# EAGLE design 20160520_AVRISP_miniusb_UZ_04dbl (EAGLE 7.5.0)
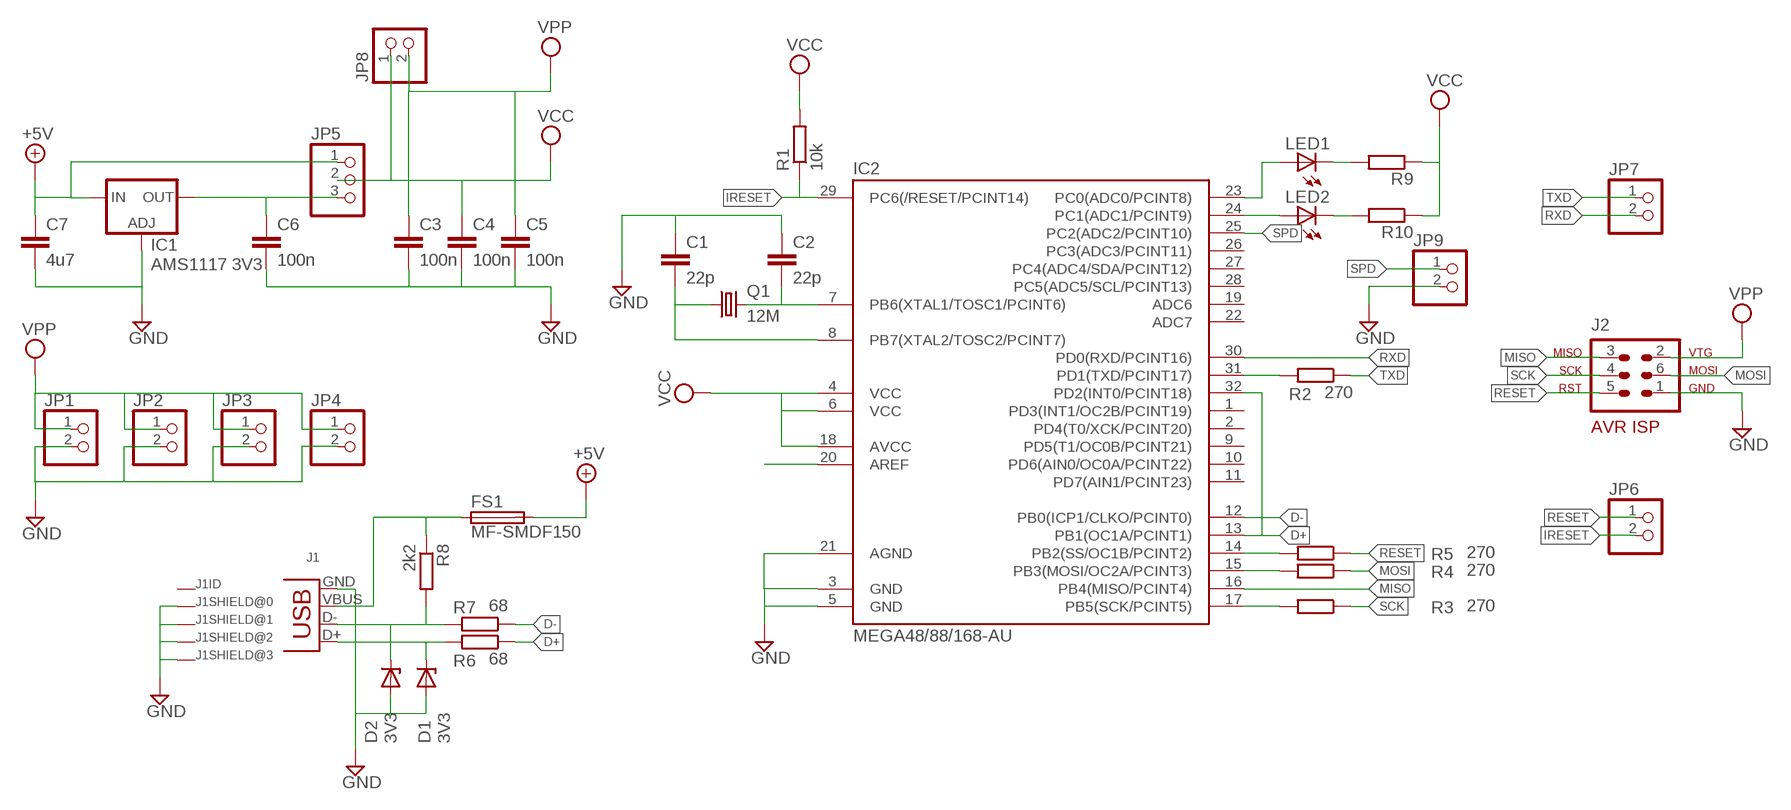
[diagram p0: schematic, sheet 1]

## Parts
C1  22p  C-EUC0805  [C0805]
C2  22p  C-EUC0805  [C0805]
C3  100n  C-EUC0805  [C0805]
C4  100n  C-EUC0805  [C0805]
C5  100n  C-EUC0805  [C0805]
C6  100n  C-EUC0805  [C0805]
C7  4u7  C-EUC1206  [C1206]
D1  3V3  ZENER-DIODESOD80C  [SOD80C]
D2  3V3  ZENER-DIODESOD80C  [SOD80C]
FS1  MF-SMDF150  [MF-SMDF050]
IC1  AMS1117 3V3  LD117AS33TR  [SOT223]
IC2  MEGA48/88/168-AU  [TQFP32-08]
J1  MINIUSB_SHIELD  [USB-MB-S2]
J2  AVR-ISP-6SPARKFUN  [SIL06]
JP1  PINHD-1X2  [1X02]
JP2  PINHD-1X2  [1X02]
JP3  PINHD-1X2  [1X02]
JP4  PINHD-1X2  [1X02]
JP5  PINHD-1X3  [1X03]
JP6  PINHD-1X2  [1X02]
JP7  PINHD-1X2  [1X02]
JP8  PINHD-1X2  [1X02]
JP9  PINHD-1X2  [1X02]
LED1  LEDCHIP-LED0805  [CHIP-LED0805]
LED2  LEDCHIP-LED0805  [CHIP-LED0805]
Q1  12M  CRYSTALHC49U-V  [HC49U-V]
R1  10k  R-EU_M0805  [M0805]
R2  270  R-EU_M0805  [M0805]
R3  270  R-EU_M0805  [M0805]
R4  270  R-EU_M0805  [M0805]
R5  270  R-EU_M0805  [M0805]
R6  68  R-EU_M0805  [M0805]
R7  68  R-EU_M0805  [M0805]
R8  2k2  R-EU_M0805  [M0805]
R9  R-EU_M0805  [M0805]
R10  R-EU_M0805  [M0805]

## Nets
+5V: C7.1 FS1.2 IC1.3(IN) JP5.1
D+: IC2.13(PB1(OC1A/PCINT1)) IC2.32(PD2(INT0/PCINT18)) R6.1
D-: IC2.12(PB0(ICP1/CLKO/PCINT0)) R7.1
GND: C1.1 C2.1 C3.2 C4.2 C5.2 C6.2 C7.2 D1.A D2.A IC1.1(ADJ) IC2.3(GND) IC2.5(GND) IC2.21(AGND) J1.GND J1.P$1(P) J1.P$2(P) J1.P$3(P) J1.P$4(P) J2.1(GND) JP1.2 JP2.2 JP3.2 JP4.2 JP9.2
IRESET: IC2.29(PC6(/RESET/PCINT14)) JP6.2 R1.1
LED1: LED1.C R9.2
MISO: IC2.16(PB4(MISO/PCINT4)) J2.3(MISO)
MOSI: J2.6(MOSI) R4.1
N$1: C2.2 IC2.7(PB6(XTAL1/TOSC1/PCINT6)) Q1.2
N$2: C1.2 IC2.8(PB7(XTAL2/TOSC2/PCINT7)) Q1.1
N$3: IC2.23(PC0(ADC0/PCINT8)) LED1.A
N$5: IC2.24(PC1(ADC1/PCINT9)) LED2.A
N$6: LED2.C R10.2
N$7: FS1.1 J1.VBUS R8.1
N$9: D2.C J1.D- R7.2 R8.2
N$10: D1.C J1.D+ R6.2
N$13: IC2.20(AREF)
N$16: IC2.31(PD1(TXD/PCINT17)) R2.2
N$17: IC2.14(PB2(SS/OC1B/PCINT2)) R5.2
N$18: IC2.15(PB3(MOSI/OC2A/PCINT3)) R4.2
N$19: IC2.17(PB5(SCK/PCINT5)) R3.2
N$22: C6.1 IC1.4(OUT) JP5.3
RESET: J2.5(RST) JP6.1 R5.1
RXD: IC2.30(PD0(RXD/PCINT16)) JP7.2
SCK: J2.4(SCK) R3.1
SPD: IC2.25(PC2(ADC2/PCINT10)) JP9.1
TXD: JP7.1 R2.1
VCC: C4.1 IC2.4(VCC) IC2.6(VCC) IC2.18(AVCC) JP5.2 JP8.1 R1.2 R9.1 R10.1
VPP: C3.1 C5.1 J2.2(VTG) JP1.1 JP2.1 JP3.1 JP4.1 JP8.2
Unconnected: IC2.1(PD3(INT1/OC2B/PCINT19)) IC2.2(PD4(T0/XCK/PCINT20)) IC2.9(PD5(T1/OC0B/PCINT21)) IC2.10(PD6(AIN0/OC0A/PCINT22)) IC2.11(PD7(AIN1/PCINT23)) IC2.19(ADC6) IC2.22(ADC7) IC2.26(PC3(ADC3/PCINT11)) IC2.27(PC4(ADC4/SDA/PCINT12)) IC2.28(PC5(ADC5/SCL/PCINT13)) J1.ID(P)

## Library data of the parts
C1-C7 = rcl:C-EU: CAPACITOR, European symbol
D1 D2 = diode:ZENER-DIODE: Z-Diode
FS1 = fuse:MF-SMDF: MF-SMDF Series - PRC Resettable Fuses
IC1 = v-reg:LD117A?*: Low drop fixed and adjustable positive voltage regulators 1 A Source: http://www.st.com/stonline/products/literature/ds/7194/ld1117axx.pdf
IC2 = avr-4:MEGA48/88/168
J1 = con-usb-3:MINIUSB_SHIELD
J2 = avr-4:AVR-ISP-6: AVR ISP-6 Serial Programming Header
JP1-JP4 JP6-JP9 = pinhead:PINHD-1X2: PIN HEADER
JP5 = pinhead:PINHD-1X3: PIN HEADER
LED1 LED2 = led:LED: LED
Q1 = crystal:CRYSTAL: CRYSTAL; OC_FARNELL: 1666969; OC_NEWARK: unknown
R1-R10 = rcl:R-EU_: RESISTOR, European symbol

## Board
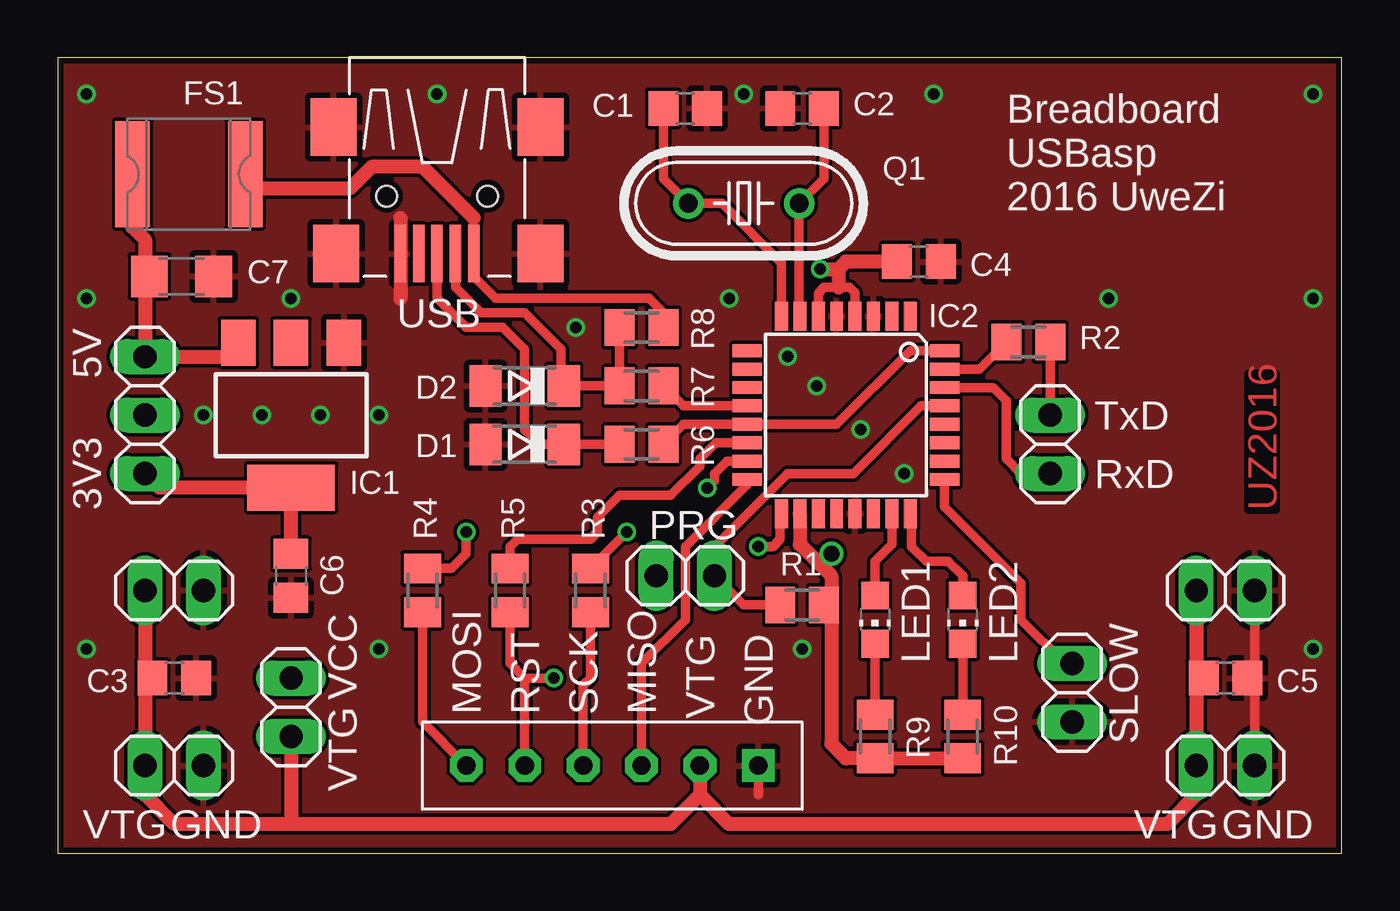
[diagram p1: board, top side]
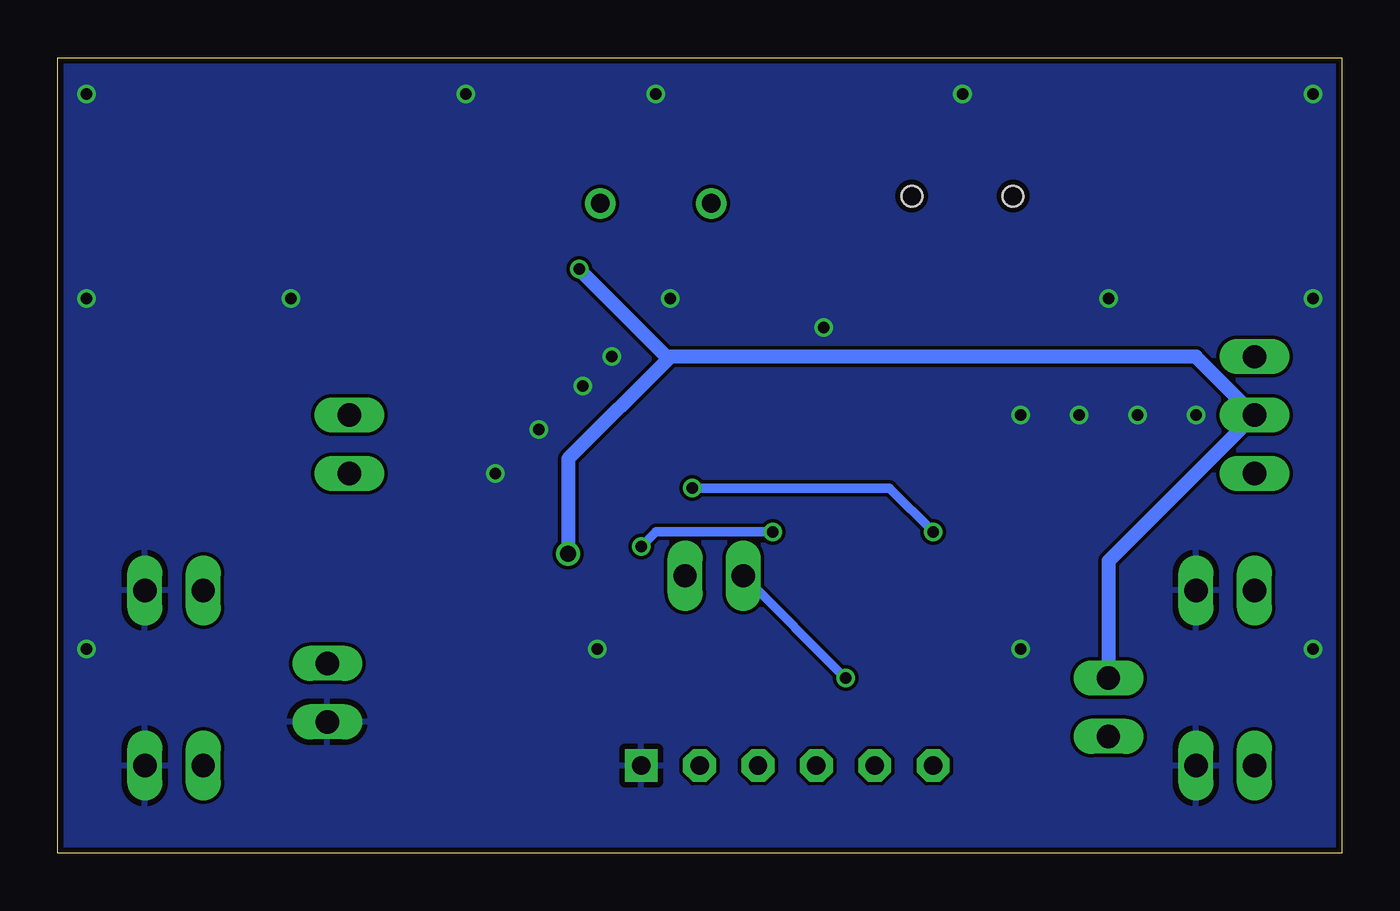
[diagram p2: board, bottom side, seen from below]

Size 55.87 x 34.6 mm. Coordinates in mm from the lower left corner, seen from the top.
Outline: 0,0 55.87,0 55.87,34.6 0,34.6 0,0
Copper layers (1*16): Top 0.035mm / dielectric 1.5mm / Bottom 0.035mm
Design rules "SeeedStudio_2layer_DRU_no_angle_20140221_02": minimum track width 6mil, minimum drill 12mil, track to track 6mil, track to pad 6mil, pad to pad 6mil, via to via 6mil, smd to smd 0mil, copper to edge 10mil, drill to drill 10mil, minimum pad ring 10mil, minimum via ring 6mil, stop-mask expansion 2mil, vias tented up to drill 100mil, thermal gap 10mil

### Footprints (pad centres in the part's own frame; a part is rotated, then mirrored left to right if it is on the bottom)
C0805 = smd 1.3 x 1.5: 1 -0.95,0; 2 0.95,0
C1206 = smd 1.6 x 1.8: 1 -1.4,0; 2 1.4,0
SOD80C = smd 1.4 x 1.8: A 1.7,0; C -1.7,0
MF-SMDF050 = smd 1.5 x 4.6: 1 -2.45,0; 2 2.45,0
SOT223 = smd 1.5 x 2: 1 -2.3,-3.15; 2 0,-3.15; 3 2.3,-3.15 | smd 3.8 x 2: 4 0,3.15
TQFP32-08 = smd 1.27 x 0.559: 1 -4.293,2.8; 2 -4.293,2; 3 -4.293,1.2; 4 -4.293,0.4; 5 -4.293,-0.4; 6 -4.293,-1.2; 7 -4.293,-2; 8 -4.293,-2.8; 17 4.293,-2.8; 18 4.293,-2; 19 4.293,-1.2; 20 4.293,-0.4; 21 4.293,0.4; 22 4.293,1.2; 23 4.293,2; 24 4.293,2.8 | smd 0.559 x 1.27: 9 -2.8,-4.293; 10 -2,-4.293; 11 -1.2,-4.293; 12 -0.4,-4.293; 13 0.4,-4.293; 14 1.2,-4.293; 15 2,-4.293; 16 2.8,-4.293; 25 2.8,4.293; 26 2,4.293; 27 1.2,4.293; 28 0.4,4.293; 29 -0.4,4.293; 30 -1.2,4.293; 31 -2,4.293; 32 -2.8,4.293
USB-MB-S2 = smd 2.5 x 0.5: D+ 2.5,0; D- 2.5,0.8; GND 2.5,-1.6; ID 2.5,-0.8; VBUS 2.5,1.6 | smd 2.5 x 2: P$1 -3,-4.5; P$2 -3,4.5; P$3 2.5,-4.4; P$4 2.5,4.5 | hole 0.9: 0,2.2; 0,-2.2
SIL06 = drill 0.8 pad 1.422 square: 1 0,0 | drill 0.8 pad 1.422 octagon: 2 2.54,0; 3 5.08,0; 4 7.62,0; 5 10.16,0; 6 12.7,0
1X02 = drill 1.016 long: 1 -1.27,0; 2 1.27,0
1X03 = drill 1.016 long: 1 -2.54,0; 2 0,0; 3 2.54,0
CHIP-LED0805 = smd 1.2 x 1.2: A 0,-1.05; C 0,1.05
HC49U-V = drill 0.813: 1 -2.413,0; 2 2.413,0
M0805 = smd 1.3 x 1.6: 1 -0.95,0; 2 0.95,0

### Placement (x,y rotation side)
C1  27.3,32.38 180 top
C2  32.38,32.38 0 top
C3  5.08,7.62 0 top
C4  37.47,25.72 0 top
C5  50.8,7.62 0 top
C6  10.16,12.06 270 top
C7  5.4,25.08 0 top
D1  20.32,17.78 180 top
D2  20.32,20.32 180 top
FS1  5.71,29.53 180 top
IC1  10.16,19.05 180 top
IC2  34.29,19.05 270 top
J1  16.51,28.57 270 top
J2  30.48,3.81 180 top
JP1  5.08,3.81 0 top
JP2  5.08,11.43 0 top
JP3  50.8,3.81 0 top
JP4  50.8,11.43 0 top
JP5  3.81,19.05 270 top
JP6  27.3,12.06 0 top
JP7  43.18,17.78 270 top
JP8  10.16,6.35 270 top
JP9  44.13,6.99 270 top
LED1  35.56,10.16 180 top
LED2  39.37,10.16 180 top
Q1  29.84,28.26 0 top
R1  32.38,10.79 0 top
R2  42.23,22.23 180 top
R3  23.18,11.43 90 top
R4  15.88,11.43 90 top
R5  19.68,11.43 90 top
R6  25.4,17.78 180 top
R7  25.4,20.32 180 top
R8  25.4,22.86 180 top
R9  35.56,5.08 90 top
R10  39.37,5.08 90 top

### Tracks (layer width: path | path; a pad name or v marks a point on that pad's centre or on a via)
+5V
  Top 0.61: IC1.3 7.25,21.59 JP5.1 3.81,25.27 | FS1.2 3.27,27.21 3.81,26.67 3.81,25.27 | 3.81,25.27 C7.1
D+
  Top 0.406: R6.1 27.22,18.65 IC2.13 33.89,18.65 37.09,21.85 IC2.32
D-
  Top 0.406: IC2.12 27.22,19.45 R7.1
GND  (via drill 0.5)
  Top 0.406: 12.7,22.86 12.7,22.44 IC1.1 | JP4.2 52.07,7.62 | 52.07,7.62 JP3.2 | C5.2 52.07,7.62 | 33.97,23.43 IC2.5 | J2.1 30.48,2.54
  Top 0.61: 14.92,27.62 14.92,24.13
  other vias: 16.51,33.02 31.75,21.59 36.83,16.51 22.54,22.86 13.97,8.89 32.38,8.89 45.72,24.13 29.21,24.13 54.61,24.13 1.27,24.13 38.1,33.02 29.84,33.02 1.27,33.02 54.61,33.02 11.43,19.05 8.89,19.05 13.97,19.05 6.35,19.05 10.16,24.13 34.92,18.41 33.02,20.32 1.27,8.89 54.61,8.89
  pour Top: 0,0 0,34.61 55.88,34.61 55.88,0
  pour Bottom: 0,0 0,34.61 55.88,34.61 55.88,0
IRESET
  Top 0.406: IC2.29 37.55,19.45 34.61,16.51 31.75,16.51 28.57,13.34 JP6.2 29.84,10.79 R1.1
LED1
  Top 0.406: LED1.C R9.2
MISO
  Top 0.406: IC2.16 30,16.03 27.3,13.34 27.3,10.16 25.4,8.26 J2.3
MOSI
  Top 0.406: R4.1 15.88,5.71 J2.6
N$1
  Top 0.406: C2.2 33.34,29.33 Q1.2 32.26,23.38 IC2.7
N$2
  Top 0.406: C1.2 26.36,29.33 Q1.1 28.89,28.26 31.49,25.66 IC2.8
N$3
  Top 0.406: IC2.23 36.29,13.43 35.56,12.7 LED1.A
N$5
  Top 0.406: IC2.24 37.15,14.76 37.15,13.34 37.78,12.7 38.73,12.7 39.37,12.06 LED2.A
N$6
  Top 0.406: LED2.C R10.2
N$7
  Top 0.406: R8.1 26.35,23.5 25.72,24.13 19.05,24.13 18.11,25.07 J1.VBUS 18.1,26.09 18.1,27.62
  Top 0.61: 18.1,27.62 15.88,29.84 13.65,29.84 12.7,28.89 8.8,28.89 FS1.1 8.48,29.84
N$9
  Top 0.406: R8.2 R7.2 D2.C 21.91,20.43 21.91,21.91 20.32,23.5 18.41,23.5 17.31,24.6 J1.D-
N$10
  Top 0.406: R6.2 D1.C 20.95,17.78 20.32,18.41 20.32,21.91 19.37,22.86 17.78,22.86 16.51,24.13 J1.D+
N$16
  Top 0.406: IC2.31 40.1,21.05 R2.2
N$17
  Top 0.406: IC2.14 28.64,17.85 27.94,17.14 27.94,16.83 26.67,15.56 24.45,15.56 23.5,14.61 23.5,13.97 23.18,13.65 20,13.65 19.68,13.34 R5.2
N$18  (via drill 0.5)
  Top 0.406: IC2.15 29.11,17.05 28.57,16.51 28.57,16.19 v28.26,15.88 | v17.78,13.97 17.78,13.02 17.14,12.38 R4.2
  Bottom 0.406: v28.26,15.88 19.68,15.88 v17.78,13.97
N$19  (via drill 0.5)
  Top 0.406: R3.2 v24.77,13.97 | v30.48,13.34 31.11,13.34 31.43,13.65 31.43,14.7 IC2.17
  Bottom 0.406: v24.77,13.97 29.84,13.97 v30.48,13.34
N$22
  Top 0.61: C6.1 IC1.4 4.42,15.9 JP5.3
RESET  (via drill 0.5)
  Top 0.406: J2.5 20.32,7.62 | 20.32,7.62 19.68,8.26 R5.1 | v21.59,7.62 20.32,7.62
  Bottom 0.406: JP6.1 v21.59,7.62
RXD
  Top 0.406: IC2.30 40.71,20.25 41.27,19.68 41.27,17.14 41.91,16.51 JP7.2
SCK
  Top 0.406: J2.4 22.86,7.3 23.18,7.62 R3.1
SPD
  Top 0.406: JP9.1 43.81,8.26 41.91,10.16 41.91,11.75 38.58,15.07 IC2.25
TXD
  Top 0.406: JP7.1 43.18,21.59 R2.1
VCC  (via drill 0.5, 0.7)
  Top 0.406: 33.02,23.27 IC2.6 33.09,24.36 33.34,24.61 33.97,24.61 34.45,24.61 34.69,24.36 IC2.4 | 33.66,12.06 33.66,11.12 R1.2
  Top 0.61: 39.69,3.81 R10.1 R9.1 34.29,4.13 33.66,4.76 33.66,12.06 33.18,12.54 | 33.97,25.4 34.29,25.72 C4.1 | 33.97,25.4 33.97,24.61 | v33.18,25.4 33.97,25.4 | IC2.18 32.29,13.43 33.18,12.54 | 33.18,12.54 v33.66,13.02
  Bottom 0.61: 29.21,21.59 6.35,21.59 JP5.2 10.16,12.7 JP8.1 | 29.21,21.59 29.37,21.59 v33.18,25.4 | 29.21,21.59 33.66,17.14 v33.66,13.02
VPP
  Top 0.61: 27.94,2.54 26.67,1.27 10.16,1.27 | 10.16,1.27 5.08,1.27 3.81,2.54 JP1.1 JP2.1 3.81,7.94 C3.1 | JP8.2 10.16,1.27 | J2.2 27.94,2.54 | 27.94,2.54 29.21,1.27 48.26,1.27 49.53,2.54 JP3.1 JP4.1 49.53,7.94 C5.1

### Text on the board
Top: UZ2016
tPlace: Breadboard / USBasp / 2016 UweZi | USB | 5V | TxD | RxD | 3V3 | PRG | VTG | GND | VCC | MOSI | RST | SCK | MISO | SLOW | VTG | VTG | GND | VTG | GND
